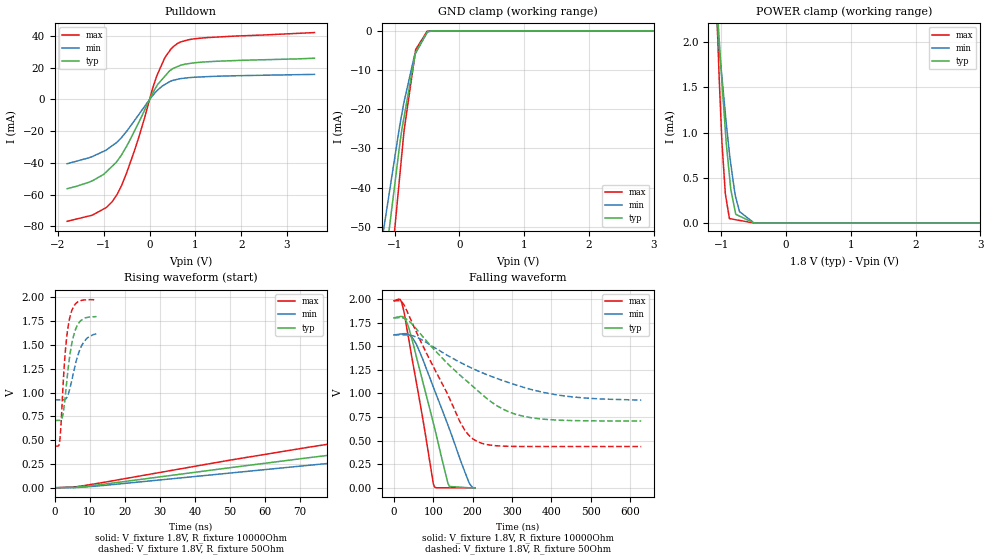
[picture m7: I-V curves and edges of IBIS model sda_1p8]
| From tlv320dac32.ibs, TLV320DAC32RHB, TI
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|   sda_1p8 Model
[Model]   sda_1p8
Model_type   I/O_open_drain
Polarity   Inverting
Vinl = 0.54
Vinh = 1.26
Vmeas = 0.9
Vref = 1.8
Cref = 10pF
Rref = 10000
|   typ   min   max
|   (nom PVT)   (fast PVT)   (slow PVT)
|C_comp from frequency sweep method (F=0.4MHz)
|C_comp   3.007e-10   2.949e-10   3.013e-10
|ON state : BUFFER OUTPUT TURNED LOW
|C_comp   5.978e-10   5.862e-10   5.989e-10
|OFF state: BUFFER IN HIGH IMPEDANCE
|C_comp   3.650e-12   3.632e-12   3.670e-12
|C_comp from LC tank measurement(L=1nH)
|Resonant Frequency(Hz)   4.520e+09   4.540e+09   4.520e+09
|C_comp   1.241e-12   1.230e-12   1.241e-12
|ON state : BUFFER OUTPUT TURNED LOW
|Resonant Frequency(Hz)   4.520e+09   4.540e+09   4.520e+09
|C_comp   1.241e-12   1.230e-12   1.241e-12
|OFF state: BUFFER IN HIGH IMPEDANCE
|Resonant Frequency(Hz)   4.630e+09   4.640e+09   4.630e+09
C_comp   1.183e-12   1.178e-12   1.183e-12
[Model spec]
|subparameter   typ   min   max
Vinl   0.54   0.486   0.594
Vinh   1.26   1.134   1.386
| Where nom  PVT is Nominal Process, 1.8V, 45C
|   Fast PVT is Strong Process,  1.98V, -40C
|   Slow PVT is Weak Process,   1.62V, 105C
[Voltage Range]   1.8   1.62   1.98
|Ambient Temperature   25   85   -40
|Junction Temperature
[Temperature Range]   45   105   -40
[Pullup Reference]   1.8   1.62   1.98
[Pulldown Reference]   0   0   0
[Power Clamp Reference]   1.8   1.62   1.98
[GND Clamp Reference]   0   0   0
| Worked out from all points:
|   slope of the pulldown table from 0 to 0.27 V, typ, clamps not added: 21.5 ohm
|   GND clamp passes 1 mA (typ) near -0.52 V on its own axis
|   POWER clamp passes 1 mA (typ) near -0.94 V on its own axis
|   falling waveform, V_fixture 1.8V, R_fixture 10000Ohm: 20-80 % time 64.9ns typ, 87.1ns min, 49.3ns max; typ from 1.8 V to 0.003 V
|   rising waveform, V_fixture 1.8V, R_fixture 10000Ohm: 20-80 % time 455ns typ, 535ns min, 374ns max; typ from 0.003 V to 1.8 V
|   falling waveform, V_fixture 1.8V, R_fixture 50Ohm: 20-80 % time 165ns typ, 223ns min, 108ns max; typ from 1.8 V to 0.709 V
|   rising waveform, V_fixture 1.8V, R_fixture 50Ohm: 20-80 % time 2.36ns typ, 3.05ns min, 1.81ns max; typ from 0.708 V to 1.8 V
[Pulldown]
|   Voltage   I(typ)   I(min)   I(max)
-1.8V     -56.25mA   -40.52mA   -76.81mA
-1.247V   -51.26mA   -35.99mA   -72.91mA
-938.5mV  -45.46mA   -31.7mA    -68mA
-708.8mV  -38.88mA   -26.81mA   -59.84mA
-495mV    -29.14mA   -19.86mA   -45.8mA
-326.7mV  -19.69mA   -13.17mA   -32.01mA
160.4mV   8.697mA    5.502mA    15.11mA
348.5mV   15.15mA    9.703mA    26.97mA
601.9mV   20.64mA    12.68mA    35.19mA
855.4mV   22.62mA    13.75mA    37.7mA
1.277V    23.8mA     14.43mA    39.06mA
3.6V      26.01mA    15.83mA    42.19mA
[GND Clamp]
|   Voltage   I(typ)   I(min)   I(max)
-1.8V     -222.1mA   -132.7mA   -331mA
-1.166V   -62.3mA    -50.46mA   -81.31mA
-1.129V   -56.81mA   -46.43mA   -73.55mA
-923.4mV  -29.45mA   -24.53mA   -37.73mA
-885.6mV  -25mA      -21.06mA   -31.13mA
-853.4mV  -22.01mA   -18.14mA   -25.55mA
-690.1mV  -6.889mA   -6.13mA    -6.698mA
-673.2mV  -5.484mA   -5.632mA   -4.744mA
-495mV    -240.3uA   -381.4uA   -65.71uA
-426.1mV  -44.37uA   -83.05uA   -6.449uA
-307.8mV  -1.264uA   -4.601uA   -85.81nA
3.6V      0A         0A         0A
[POWER Clamp]
|   Voltage   I(typ)   I(min)   I(max)
-1.8V     11.87mA    8.619mA    19.35mA
-1.085V   2.649mA    2.361mA    2.616mA
-1.039V   2.086mA    1.979mA    1.704mA
-990mV    1.542mA    1.604mA    881.4uA
-938.5mV  1.023mA    1.21mA     323.2uA
-923.4mV  874.4uA    1.094mA    257.8uA
-875.2mV  522uA      770.1uA    49.36uA
-855mV    374.8uA    656.9uA    46.74uA
-777.6mV  96.52uA    281.9uA    36.69uA
-719.3mV  76.6uA     126.4uA    29.12uA
-494.1mV  11.68nA    505.4nA    0A
3.6V      0A         0A         0A
[Ramp]
R_load = 10000
|   typ   min   max
dV/dt_r   1.07775/4.53941e-07   0.968003/5.34094e-07   1.18683/3.72886e-07
dV/dt_f   1.07828/6.4781e-08   0.969552/8.68324e-08   1.18693/4.92847e-08
[Falling Waveform]
V_fixture = 1.8V
V_fixture_min = 1.62V
V_fixture_max = 1.98V
R_fixture = 10000Ohm
|   Time   V(typ)   V(min)   V(max)
0s        1.8V       1.62V      1.98V
15.7ns    1.814V     1.628V     1.994V
24.4ns    1.806V     1.632V     1.883V
36.6ns    1.707V     1.625V     1.598V
55.3ns    1.418V     1.533V     1.154V
102.2ns   652.7mV    1.045V     21.09mV
137ns     53.17mV    667.7mV    2.16mV
140.9ns   16.4mV     624.4mV    2.068mV
190.9ns   2.407mV    55.93mV    1.761mV
205.8ns   3.243mV    1.638mV    1.76mV
[Rising Waveform]
V_fixture = 1.8V
V_fixture_min = 1.62V
V_fixture_max = 1.98V
R_fixture = 10000Ohm
|   Time   V(typ)   V(min)   V(max)
0s        2.866mV    4.073mV    1.782mV
128.9ns   552.5mV    425.9mV    721.3mV
190.8ns   766.5mV    602.4mV    978.5mV
257.4ns   955.8mV    763mV      1.197V
333.5ns   1.131V     915.7mV    1.39V
414ns     1.277V     1.048V     1.544V
608.1ns   1.511V     1.274V     1.769V
855.9ns   1.665V     1.438V     1.897V
1.237us   1.758V     1.552V     1.96V
2.5us     1.799V     1.617V     1.98V
[Falling Waveform]
V_fixture = 1.8V
V_fixture_min = 1.62V
V_fixture_max = 1.98V
R_fixture = 50Ohm
|   Time   V(typ)   V(min)   V(max)
0s        1.8V       1.62V      1.98V
25.5ns    1.797V     1.621V     1.936V
61.2ns    1.661V     1.589V     1.612V
169.5ns   1.188V     1.326V     688mV
188.9ns   1.118V     1.286V     564.3mV
210.9ns   1.037V     1.243V     493.3mV
277.7ns   833mV      1.135V     442.9mV
345.3ns   745.7mV    1.046V     439mV
446.7ns   714mV      967mV      438.8mV
628.6ns   708.6mV    929.7mV    438.8mV
[Rising Waveform]
V_fixture = 1.8V
V_fixture_min = 1.62V
V_fixture_max = 1.98V
R_fixture = 50Ohm
|   Time   V(typ)   V(min)   V(max)
0s        708.4mV    924.5mV    438.8mV
1.4ns     708.3mV    924.5mV    491mV
1.7ns     709.8mV    924.5mV    617.2mV
2.2ns     749.8mV    924.4mV    963.9mV
3ns       962.6mV    928.7mV    1.426V
3.7ns     1.215V     969.9mV    1.665V
4.6ns     1.463V     1.087V     1.831V
6ns       1.67V      1.314V     1.932V
7.7ns     1.761V     1.494V     1.967V
11.9ns    1.796V     1.616V     1.974V
